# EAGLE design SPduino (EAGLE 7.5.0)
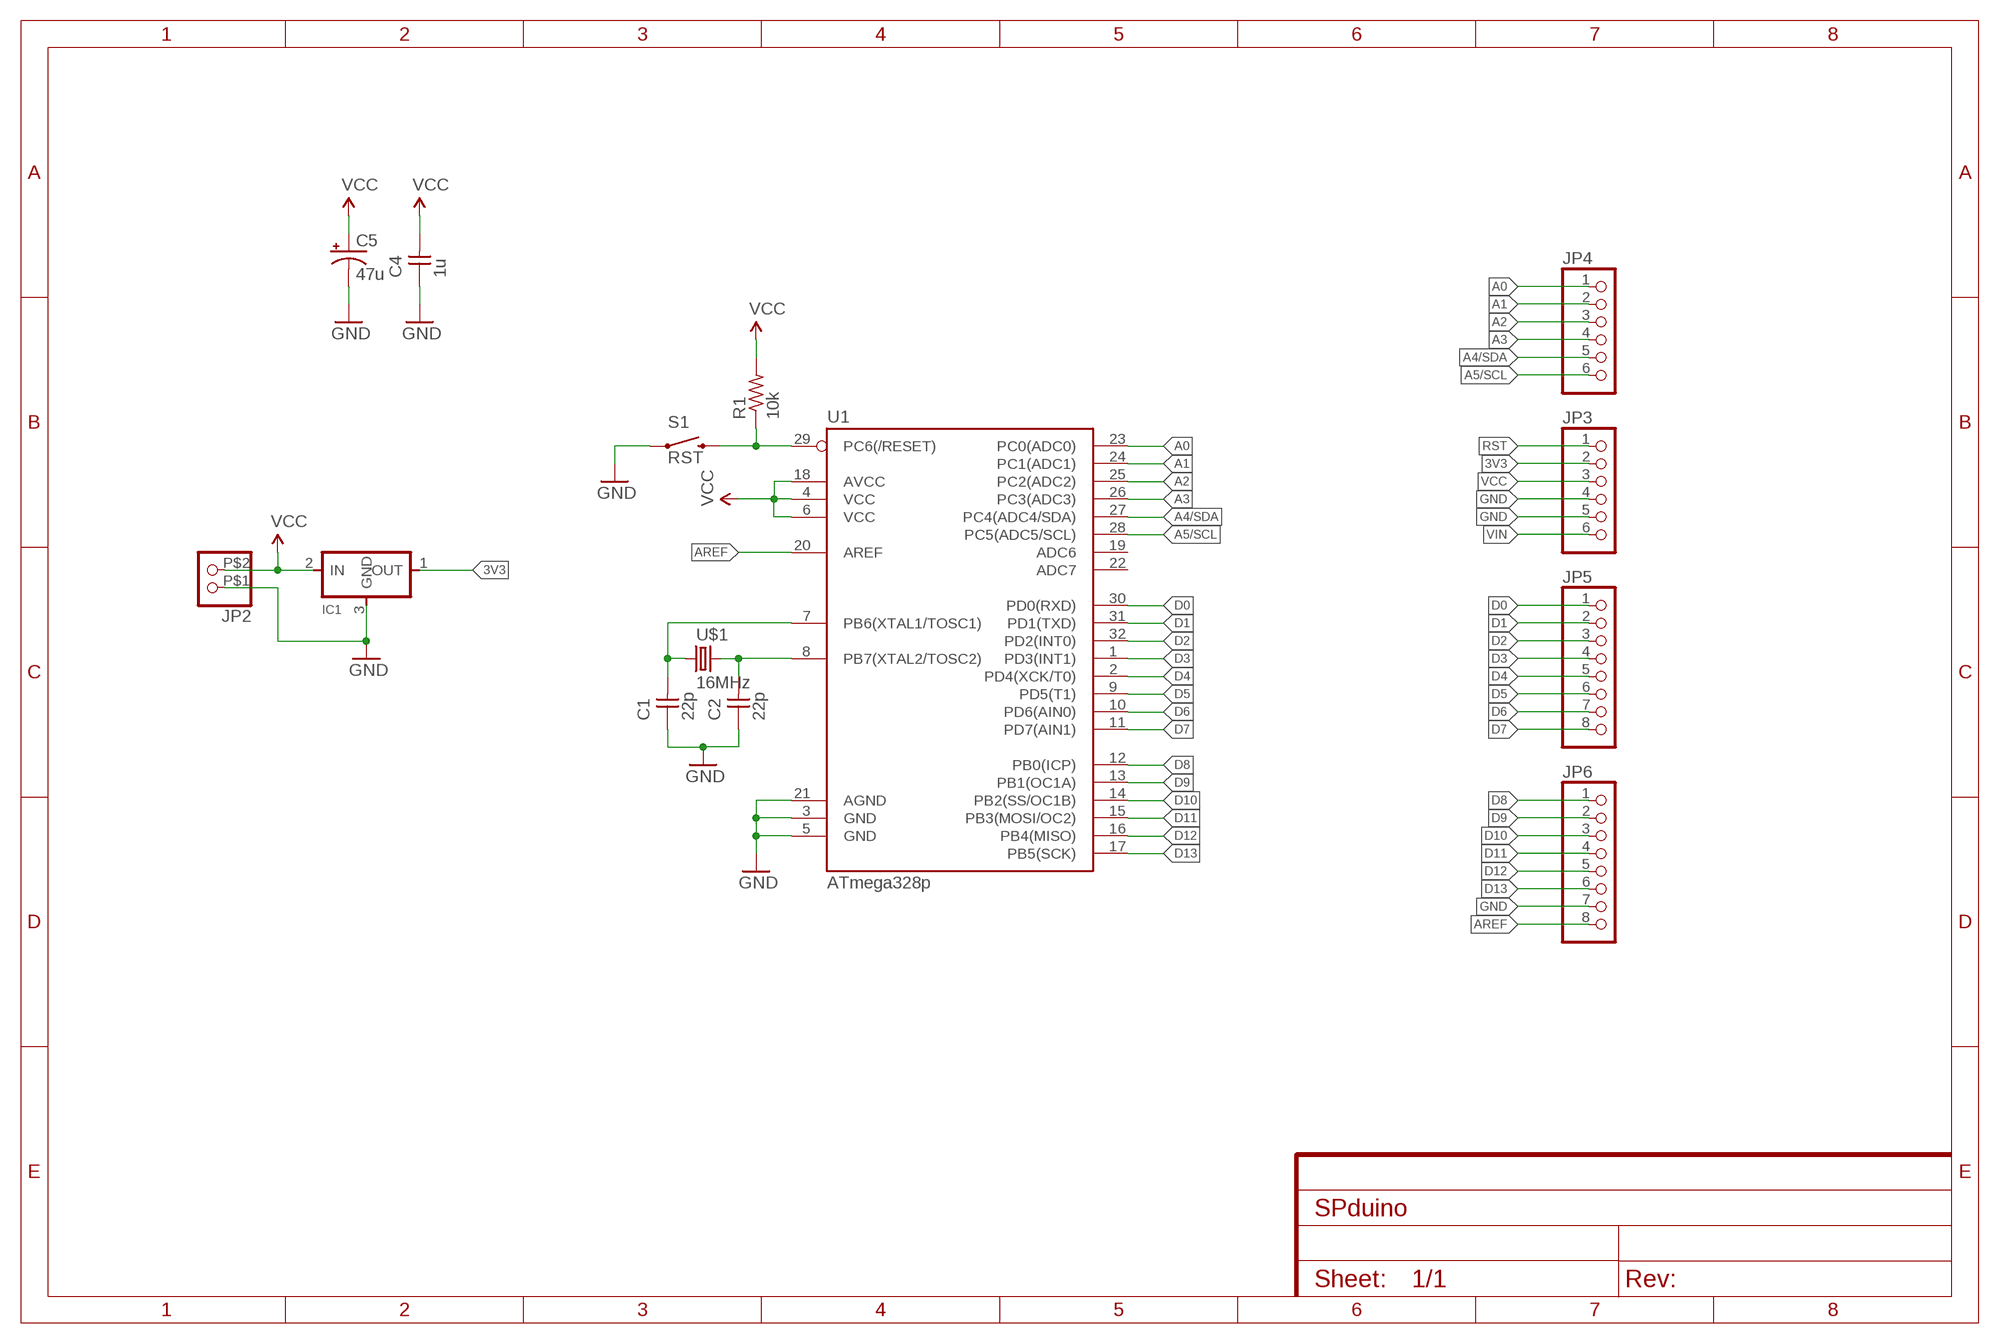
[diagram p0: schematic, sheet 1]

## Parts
C1  22p  CAP-UNPOLARIZEDFAB  [C1206FAB]
C2  22p  CAP-UNPOLARIZEDFAB  [C1206FAB]
C4  1u  CAP-UNPOLARIZEDFAB  [C1206FAB]
C5  47u  47UF-50V-20%(ELECT)  [PANASONIC_D]
IC1  REGULATORSOT23  [SOT23]
JP2  PINHD-1X2SMD  [1X02SMD]
JP3  PINHD-1X6  [1X06]
JP4  PINHD-1X6  [1X06]
JP5  PINHD-1X8  [1X08]
JP6  PINHD-1X8  [1X08]
R1  10k  RES-US1206FAB  [R1206FAB]
S1  RST  SWITCH-MOMENTARY-2SMD-6MM  [TACTILE-SMD-6MM]
U1  ATmega328p  ATMEGA328P_TQFPTQFP32-08THIN  [TQFP32-08THIN]
U$1  16MHz  CRYSTAL  [2-SMD-5X3MM]

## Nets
3V3: IC1.1(OUT) JP3.2
A0: JP4.1 U1.23(PC0(ADC0))
A1: JP4.2 U1.24(PC1(ADC1))
A2: JP4.3 U1.25(PC2(ADC2))
A3: JP4.4 U1.26(PC3(ADC3))
A4/SDA: JP4.5 U1.27(PC4(ADC4/SDA))
A5/SCL: JP4.6 U1.28(PC5(ADC5/SCL))
AREF: JP6.8 U1.20(AREF)
D0: JP5.1 U1.30(PD0(RXD))
D1: JP5.2 U1.31(PD1(TXD))
D2: JP5.3 U1.32(PD2(INT0))
D3: JP5.4 U1.1(PD3(INT1))
D4: JP5.5 U1.2(PD4(XCK/T0))
D5: JP5.6 U1.9(PD5(T1))
D6: JP5.7 U1.10(PD6(AIN0))
D7: JP5.8 U1.11(PD7(AIN1))
D8: JP6.1 U1.12(PB0(ICP))
D9: JP6.2 U1.13(PB1(OC1A))
D10: JP6.3 U1.14(PB2(SS/OC1B))
D11: JP6.4 U1.15(PB3(MOSI/OC2))
D12: JP6.5 U1.16(PB4(MISO))
D13: JP6.6 U1.17(PB5(SCK))
GND: C1.1 C2.1 C4.1 C5.- IC1.3(GND) JP2.P$1 JP3.4 JP3.5 JP6.7 S1.1 U1.3(GND) U1.5(GND) U1.21(AGND)
N$1: C1.2 U1.7(PB6(XTAL1/TOSC1)) U$1.P$1
N$2: C2.2 U1.8(PB7(XTAL2/TOSC2)) U$1.P$2
RST: JP3.1 R1.1 S1.2 U1.29(PC6(/RESET))
VCC: C4.2 C5.+ IC1.2(IN) JP2.P$2 JP3.3 R1.2 U1.4(VCC) U1.6(VCC) U1.18(AVCC)
VIN: JP3.6
Unconnected: U1.19(ADC6) U1.22(ADC7)

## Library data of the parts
C1 C2 C4 = 00fab:CAP-UNPOLARIZED
C5 = SparkFun-Capacitors:47UF-50V-20%(ELECT): CAP-10547; PROD_ID: CAP-10547
IC1 = 00fab:REGULATOR
JP2 = 00fab:PINHD-1X2: PIN HEADER
JP3 JP4 = pinhead:PINHD-1X6: PIN HEADER
JP5 JP6 = pinhead:PINHD-1X8: PIN HEADER
R1 = 00fab:RES-US: Resistor (US Symbol)
S1 = 00fab:SWITCH-MOMENTARY-2: Various NO switches- pushbuttons, reed, etc
U1 = 00fab:ATMEGA328P_TQFP
U$1 = 00fab:CRYSTAL

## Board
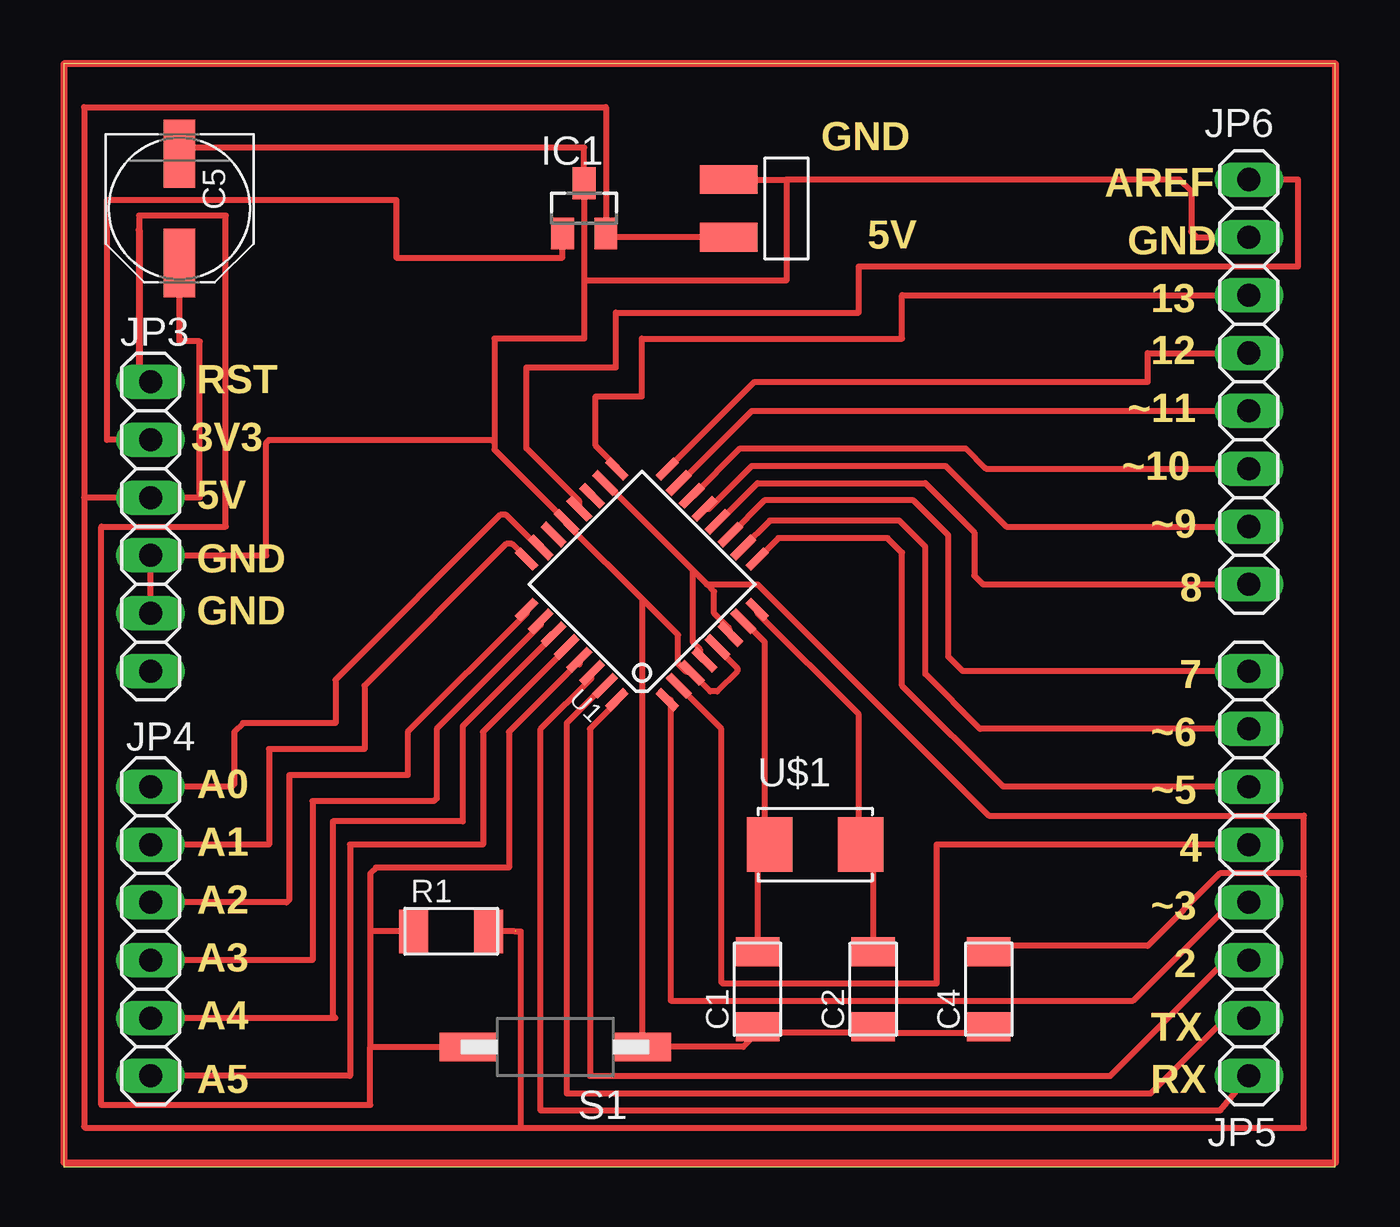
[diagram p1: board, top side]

Size 55.87 x 48.44 mm. Coordinates in mm from the lower left corner, seen from the top.
Outline: 0,48.44 0,0 55.87,0 55.87,48.44 0,48.44
Copper layers (1*16): Top 0.035mm / dielectric 1.5mm / Bottom 0.035mm
Design rules "default": minimum track width 10mil, minimum drill 24mil, track to track 8mil, track to pad 8mil, pad to pad 8mil, via to via 8mil, smd to smd 8mil, copper to edge 40mil, drill to drill 8mil, minimum pad ring 10mil, minimum via ring 8mil, stop-mask expansion 4mil, vias tented up to drill 0mil, thermal gap 10mil

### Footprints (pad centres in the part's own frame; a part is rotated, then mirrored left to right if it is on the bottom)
C1206FAB = smd 1.27 x 1.905: 1 -1.651,0; 2 1.651,0
PANASONIC_D = smd 3 x 1.4: + 2.4,0; - -2.4,0
SOT23 = smd 1 x 1.4: 1 -0.95,-1.1; 2 0.95,-1.1; 3 0,1.1
1X02SMD = smd 2.54 x 1.27: P$1 0,1.27; P$2 0,-1.27
1X06 = drill 1.016 long: 1 -6.35,0; 2 -3.81,0; 3 -1.27,0; 4 1.27,0; 5 3.81,0; 6 6.35,0
1X08 = drill 1.016 long: 1 -8.89,0; 2 -6.35,0; 3 -3.81,0; 4 -1.27,0; 5 1.27,0; 6 3.81,0; 7 6.35,0; 8 8.89,0
R1206FAB = smd 1.27 x 1.905: 1 -1.651,0; 2 1.651,0
TACTILE-SMD-6MM = smd 2.54 x 1.27: 1 -3.81,0; 2 3.81,0
TQFP32-08THIN = smd 1.118 x 0.356: 1 -4.369,2.8; 8 -4.369,-2.8; 17 4.369,-2.8; 24 4.369,2.8 | smd 1.27 x 0.356: 2 -4.293,2; 3 -4.293,1.2; 4 -4.293,0.4; 5 -4.293,-0.4; 6 -4.293,-1.2; 7 -4.293,-2; 18 4.293,-2; 19 4.293,-1.2; 20 4.293,-0.4; 21 4.293,0.4; 22 4.293,1.2; 23 4.293,2 | smd 0.356 x 1.118: 9 -2.8,-4.369; 16 2.8,-4.369; 25 2.8,4.369; 32 -2.8,4.369 | smd 0.356 x 1.27: 10 -2,-4.293; 14 1.2,-4.293; 15 2,-4.293; 26 2,4.293; 27 1.2,4.293; 31 -2,4.293 | smd 0.35 x 1.27: 11 -1.2,-4.293; 12 -0.4,-4.293; 13 0.4,-4.293; 28 0.4,4.293; 29 -0.4,4.293; 30 -1.2,4.293
2-SMD-5X3MM = smd 2 x 2.4: P$1 -2,0; P$2 2,0

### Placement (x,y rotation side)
C1  30.48,7.8 90 top
C2  35.56,7.8 90 top
C4  40.64,7.8 90 top
C5  5.08,42.09 270 top
IC1  22.86,42.09 0 top
JP2  29.21,42.09 0 top
JP3  3.81,28.12 270 top
JP4  3.81,10.34 270 top
JP5  52.07,12.88 90 top
JP6  52.07,34.47 90 top
R1  17.02,10.34 0 top
S1  21.59,5.26 180 top
U1  25.4,25.58 135 top
U$1  33.02,14.15 0 top

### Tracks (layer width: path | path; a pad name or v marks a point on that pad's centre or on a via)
3V3
  Top 0.254: JP3.2 1.91,31.93 1.91,42.47 14.61,42.47 14.61,39.93 21.91,39.93 IC1.1
A0
  Top 0.254: U1.23 20.86,27.2 19.43,28.63 19.18,28.63 11.94,21.39 11.94,19.48 7.87,19.48 7.49,19.1 7.49,16.82 7.37,16.69 JP4.1
A1
  Top 0.254: U1.24 20.33,26.71 19.68,27.36 19.43,27.36 13.21,21.13 13.21,18.34 9.02,18.34 9.02,14.15 JP4.2
A2
  Top 0.254: U1.25 20.33,24.32 15.11,19.1 15.11,17.2 9.91,17.2 9.91,11.74 9.78,11.61 JP4.3
A3
  Top 0.254: U1.26 20.95,23.8 16.38,19.23 16.38,16.18 16.26,16.05 10.92,16.05 10.92,9.07 JP4.4
A4/SDA
  Top 0.254: U1.27 21.52,23.35 17.53,19.36 17.53,15.16 11.81,15.16 11.81,6.66 11.94,6.53 JP4.5
A5/SCL
  Top 0.254: U1.28 22.08,22.77 18.41,19.1 18.41,14.15 12.57,14.15 12.57,3.99 JP4.6
AREF
  Top 0.254: U1.20 22.65,29.22 20.32,31.55 20.32,35.1 24.26,35.1 24.26,37.52 34.92,37.52 34.92,39.55 54.23,39.55 54.23,43.36 JP6.8
D0
  Top 0.254: JP5.1 50.8,2.46 20.95,2.46 20.95,19.23 23.18,21.45 U1.30
D1
  Top 0.254: U1.31 23.74,21.13 22.1,19.48 22.1,3.23 47.75,3.23 51.05,6.53 JP5.2
D2
  Top 0.254: U1.32 24.29,20.41 23.11,19.23 23.11,3.99 45.97,3.99 51.05,9.07 JP5.3
D3
  Top 0.254: U1.1 26.67,20.5 26.67,7.29 46.99,7.29 51.31,11.61 JP5.4
D4
  Top 0.254: JP5.5 38.35,14.15 38.35,8.05 28.96,8.05 28.89,8.12 28.89,19.23 27.3,20.82 U1.2
D5
  Top 0.254: JP5.6 41.27,16.69 36.83,21.13 36.83,26.98 36.2,27.61 31.39,27.61 U1.9
D6
  Top 0.254: JP5.7 40.26,19.23 37.85,21.64 37.85,27.23 36.7,28.37 31.02,28.37 U1.10
D7
  Top 0.254: JP5.8 39.5,21.77 38.86,22.4 38.86,27.74 37.34,29.26 30.78,29.26 U1.11
D8
  Top 0.254: U1.12 28.79,28.33 30.48,30.02 37.85,30.02 40.01,27.86 40.01,25.96 40.39,25.58 JP6.1
D9
  Top 0.254: U1.13 28.34,28.9 30.23,30.79 38.73,30.79 41.4,28.12 JP6.2
D10
  Top 0.254: U1.14 27.63,29.46 29.72,31.55 39.62,31.55 40.51,30.66 JP6.3
D11
  Top 0.254: U1.15 27.06,30.03 30.23,33.2 JP6.4
D12
  Top 0.254: U1.16 26.53,30.65 30.35,34.47 47.62,34.47 47.62,35.74 JP6.5
D13
  Top 0.254: U1.17 24.29,30.75 23.37,31.67 23.37,33.83 25.4,33.83 25.4,36.37 36.83,36.37 36.83,38.28 JP6.6
GND
  Top 0.254: 31.75,43.36 49.02,43.36 49.53,42.85 49.53,41.07 49.78,40.82 JP6.7 | 5.08,44.31 C5.- 5.08,44.75 22.86,44.75 IC1.3 22.86,38.91 | 35.56,5.89 30.48,5.89 | 35.56,5.89 40.64,5.89 C4.1 | 35.56,5.89 C2.1 | 30.48,5.89 29.84,5.26 S1.1 25.4,24.94 | 30.48,5.89 C1.1 | JP3.5 JP3.4 8.89,26.85 8.89,31.8 9.02,31.93 18.8,31.93 18.92,31.8 | 25.4,24.94 26.99,23.36 26.99,22.09 27.3,21.77 U1.3 28.4,20.88 28.7,20.88 29.59,21.77 29.59,21.89 28.72,22.77 U1.5 | 25.4,24.94 22.23,28.12 U1.21 18.92,31.49 18.92,31.8 | 22.86,38.91 22.86,36.37 18.92,36.37 18.92,31.8 | JP2.P$1 31.75,43.36 | 31.75,43.36 31.75,38.91 22.86,38.91
N$1
  Top 0.254: 30.8,14.15 30.8,23.04 30.16,23.67 U1.7 | C1.2 30.48,13.83 30.8,14.15 | 30.8,14.15 U$1.P$1
N$2
  Top 0.254: U1.8 30.48,24.31 34.92,19.86 34.92,14.15 U$1.P$2 35.24,14.15 35.56,13.83 C2.2
N$3
  Top 0.305: 0,0.18 55.88,0.18 55.88,48.44 0,48.44 0,0.18
RST
  Top 0.254: 3.3,41.14 3.3,41.77 7.11,41.77 7.11,28.12 1.65,28.12 1.65,2.72 13.46,2.72 13.46,5.26 | S1.2 17.4,4.88 17.02,5.26 13.46,5.26 | U1.29 22.65,22.06 22.52,22.06 19.56,19.1 19.56,13.13 13.72,13.13 13.46,12.88 13.46,10.34 | R1.1 13.46,10.34 | 13.46,10.34 13.46,5.26
  Top 0.305: 3.3,41.14 3.3,34.98 JP3.1
VCC  (1 unrouted)
  Top 0.254: 28.26,25.58 28.57,25.26 28.57,24.31 29.21,23.67 U1.6 | 28.26,25.58 27.62,26.21 | 27.62,26.21 23.81,30.02 U1.18 | 27.62,26.21 27.62,23.04 27.94,22.72 27.94,22.4 U1.4 | 28.26,25.58 30.48,25.58 40.64,15.42 54.48,15.42 54.48,12.75 | C4.2 40.64,9.7 47.62,9.7 50.8,12.88 54.36,12.88 54.48,12.75 | JP2.P$2 23.81,40.82 IC1.2 23.81,41.14 23.81,46.53 0.89,46.53 0.89,29.39 | 0.89,29.39 0.89,1.76 0.95,1.7 2.03,1.7 20.07,1.7 | 19.81,10.34 R1.2 | C5.+ 5.08,36.25 5.97,36.25 5.97,29.39 JP3.3 0.89,29.39 | 54.48,12.75 54.48,1.7 20.07,1.7 | 19.88,10.34 20.07,10.34 20.07,1.7

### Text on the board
Dimension: GND | AREF | 5V | GND | 13 | 12 | RST | ~11 | 3V3 | ~10 | 5V | ~9 | GND | 8 | GND | 7 | ~6 | A0 | ~5 | A1 | 4 | A2 | ~3 | A3 | 2 | A4 | TX | A5 | RX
